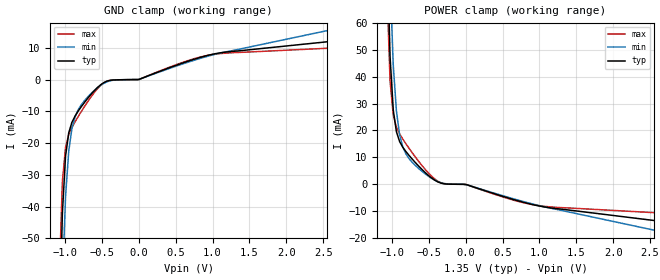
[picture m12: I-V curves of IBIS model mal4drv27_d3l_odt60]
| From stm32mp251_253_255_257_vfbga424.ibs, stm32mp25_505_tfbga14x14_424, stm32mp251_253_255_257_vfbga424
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[Model] mal4drv27_d3l_odt60
Model_type   Input
Polarity   Non-Inverting
Enable   Active-High
C_comp   1.746pF   1.678pF   1.772pF
C_comp_pullup   865.131fF   816.376fF   879.171fF
C_comp_pulldown   744.080fF   743.722fF   746.114fF
Vinh = 805.000mV
Vinl = 545.000mV
[Model Spec]
D_overshoot_ampl_h 0.4 NA   NA
D_overshoot_ampl_l 0.4 NA   NA
D_overshoot_area_l 110.000m NA   NA
D_overshoot_area_h 110.000m NA   NA
[Temperature Range]   25.000   125.000   -40.000
[Voltage Range]   1.350V   1.283V   1.425V
[GND Clamp Reference]   0.00V   0.00V   0.00V
[C Comp Corner]
| variable   typ   min   max
C_comp   1.746pF   1.678pF   1.772pF
C_comp_pullup   865.131fF   816.376fF   879.171fF
C_comp_pulldown   744.080fF   743.722fF   746.114fF
[POWER Clamp Reference]   1.350V   1.283V   1.425V
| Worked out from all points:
|   GND clamp passes 1 mA (typ) near -0.48 V on its own axis
|   POWER clamp passes 1 mA (typ) near -0.38 V on its own axis
[GND Clamp]
-1.339V   -727.9mA   -688.7mA   -716.4mA
-1.079V   -81.43mA   -108.9mA   -63.04mA
-1.036V   -42.21mA   -64.14mA   -32.12mA
-993.2mV  -24.16mA   -36.99mA   -21.31mA
-950mV    -16.82mA   -22.64mA   -17.36mA
-906.8mV  -13.49mA   -15.45mA   -15.12mA
-863.6mV  -11.49mA   -11.7mA    -13.31mA
-734.1mV  -7.152mA   -6.597mA   -8.425mA
-475mV    -986.5uA   -1.211mA   -1.044mA
-600nV    -7.074uA   -5.639uA   -8.87uA
993.2mV   7.904mA    7.687mA    7.82mA
2.677V    12.16mA    15.98mA    9.966mA
[Power Clamp]
-1.327V   868.9mA    825.6mA    851.7mA
-1.068V   91.3mA     128.5mA    73mA
-1.025V   47.43mA    76.15mA    38.34mA
-981.8mV  27.63mA    44.44mA    25.79mA
-938.6mV  19.54mA    27.18mA    21.21mA
-895.5mV  15.89mA    18.41mA    18.75mA
-852.3mV  13.76mA    13.86mA    16.82mA
-679.5mV  8.008mA    6.944mA    10.06mA
-377.3mV  893.6uA    1.027mA    1.145mA
11.4mV    -105.2uA   -144.7uA   -110.7uA
1.005V    -8.088mA   -7.96mA    -7.955mA
2.689V    -13.88mA   -17.8mA    -10.73mA
